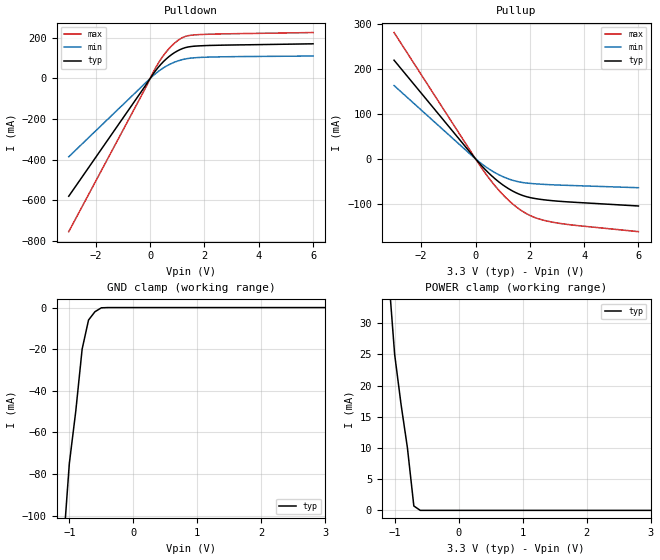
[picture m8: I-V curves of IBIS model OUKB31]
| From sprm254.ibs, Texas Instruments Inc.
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[Model]   OUKB31
Model_type   3-state
Polarity   Non-Inverting
Enable   Active-Low
| signals   A, GZ, Y
Cref = 20p
Rref = 50
Vmeas = 1.3
|   typ   min   max
C_comp   2.7937p   2.7456p   2.9292p
|   typ   min   max
[Temperature Range]   25.0   -40   125
|   typ   min   max
[Voltage Range]   3.3V   3.0V   3.6V
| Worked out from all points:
|   slope of the pulldown table from 0 to 0.495 V, typ, clamps not added: 5.92 ohm
|   slope of the pullup table from 0 to 0.495 V, typ, clamps not added: 15.4 ohm
|   GND clamp passes 1 mA (typ) near -0.55 V on its own axis
|   POWER clamp passes 1 mA (typ) near -0.70 V on its own axis
[Pulldown]
|   Voltage   I(typ)   I(min)   I(max)
-3V       -579.4mA   -385.4mA   -753.5mA
-200mV    -40.37mA   -25.84mA   -54.02mA
200mV     38.3mA     23.89mA    52.31mA
500mV     84.25mA    52.87mA    114.9mA
700mV     108.1mA    68.01mA    147.6mA
900mV     127.1mA    80.08mA    173.8mA
1.2V      147.2mA    92.87mA    201.4mA
1.6V      158.1mA    101.1mA    213.5mA
6V        170.1mA    110mA      225.5mA
[GND_clamp]
|   Voltage   I(typ)   I(min)   I(max)
-3V       -900mA     NA         NA
-2V       -500mA     NA         NA
-1V       -75mA      NA         NA
-900mV    -50mA      NA         NA
-800mV    -20mA      NA         NA
-700mV    -6mA       NA         NA
-600mV    -2mA       NA         NA
-500mV    -120uA     NA         NA
-400mV    0A         NA         NA
3V        0A         NA         NA
[Pullup]
|   Voltage   I(typ)   I(min)   I(max)
-3V       218.9mA    162.6mA    280.3mA
200mV     -13.78mA   -9.858mA   -18.22mA
500mV     -32.37mA   -22.79mA   -43.33mA
800mV     -48.41mA   -33.5mA    -65.71mA
1.1V      -61.84mA   -41.98mA   -85.23mA
1.4V      -72.6mA    -48.24mA   -101.8mA
1.7V      -80.63mA   -52.3mA    -115.3mA
2V        -85.94mA   -54.52mA   -125.6mA
2.6V      -91.55mA   -57.04mA   -137.7mA
3.5V      -96mA      -59.18mA   -146.6mA
6V        -104.7mA   -64.18mA   -161.7mA
[POWER_clamp]
|   Voltage   I(typ)   I(min)   I(max)
-3V       300mA      NA         NA
-2V       160mA      NA         NA
-1V       25mA       NA         NA
-900mV    17mA       NA         NA
-800mV    10mA       NA         NA
-700mV    700uA      NA         NA
-600mV    0A         NA         NA
-500mV    0A         NA         NA
3V        0A         NA         NA
[Ramp]
|   I(typ)   I(min)   I(max)
dV/dt_r   1.978/0.710n   1.793/1.240n   2.159/0.410n
dV/dt_f   1.980/0.650n   1.799/1.130n   2.160/0.380n
